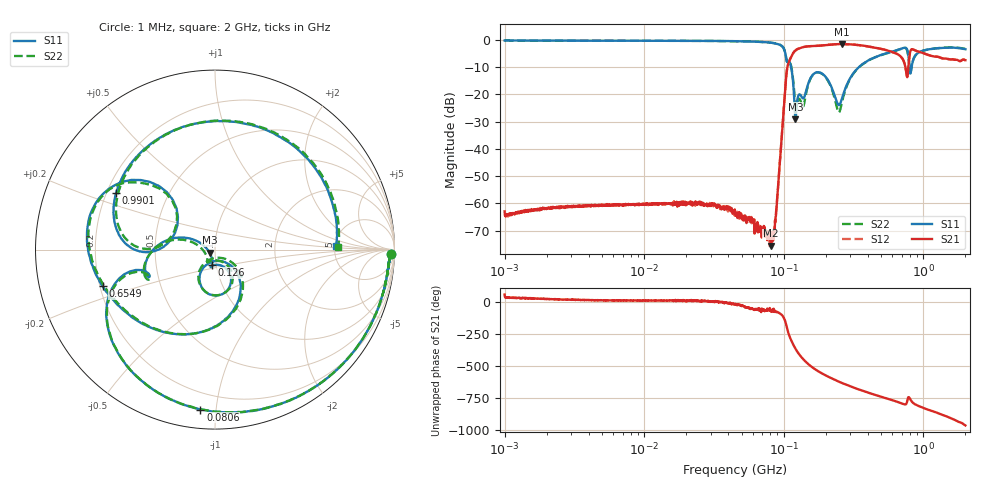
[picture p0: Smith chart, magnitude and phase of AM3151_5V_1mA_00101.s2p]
! Date/Time: Fri Jun 26 10:33:27 2020
! Network Analyzer:  Rev:
! Sweep from 1000000.0 to 2000000000.0, 1601 Points ! Power Supply: 0 V, 0 A
# HZ S DB R 50
!freq MagS11 AngS11 MagS21 AngS21 MagS12 AngS12 MagS22 AngS22
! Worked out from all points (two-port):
!   1601 points, 1 MHz to 2 GHz, reference 50 ohm
!   highest |S21| = -1.47 dB at 261.8 MHz (marker M1); lowest = -75.6 dB at 80.99 MHz (marker M2)
!   |S21| within 3 dB of the highest: 117.9 MHz to 602.8 MHz (484.9 MHz wide, 135 % of centre); 803.3 MHz to 951.4 MHz (148.1 MHz wide, 16.9 % of centre)
!   lowest |S11| = -29.2 dB at 121.3 MHz (marker M3), VSWR 1.07, Z = 47.1 - j1.64 ohm
!   |S11| at or under -10 dB: 112.9 MHz to 344.4 MHz (231.5 MHz wide, 101 % of centre); 795.6 MHz to 823.2 MHz (27.65 MHz wide, 3.42 % of centre)
!   |S22| runs from -26.6 to -0.2 dB; largest |S21 - S12| = 0.0096
!   S11 on the Smith chart (normalised r, x): 1 MHz: 37, -48; 80.6 MHz: 0.10, -0.91; 126 MHz: 0.95, -0.16; 654.9 MHz: 0.21, -0.15; 990.1 MHz: 0.24, +0.25; 2 GHz: 5.15, +0.37
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1000000  -0.17 -1.5  -62.97 59.7  -64.38 36.1  -0.17 -1.5
3555161  -0.24 -3.9  -60.89 17.4  -61.09 15.9  -0.25 -3.9
1.263916e7  -0.28 -12.7  -60.62 12.3  -60.20 12.3  -0.28 -12.7
4.493426e7  -0.43 -46.3  -63.66 -20.4  -62.81 -17.4  -0.43 -46.3
8.06017e7  -0.96 -95.2  -70.62 -68.9  -72.08 -66.7  -0.99 -95.1
8.098555e7  -0.99 -95.9  -75.59 -60.3  -74.32 -62.5  -0.99 -95.8
8.779725e7  -1.28 -109.9  -64.72 -77.8  -64.00 -72.4  -1.30 -109.7
1.051672e8  -7.85 -162.4  -11.22 162.6  -11.21 162.5  -7.81 -160.8
1.123994e8  -9.53 178.1  -6.41 66.3  -6.41 66.4  -9.15 -178.9
1.212759e8  -29.19 -150.0  -3.81 -5.8  -3.82 -5.9  -24.15 -170.7
1.259737e8  -21.19 -101.6  -3.30 -34.6  -3.30 -34.6  -22.25 -122.5
1.391892e8  -21.25 -78.8  -2.54 -92.8  -2.55 -92.7  -23.86 -72.5
1.589914e8  -13.21 -67.5  -2.23 -149.1  -2.22 -149.1  -13.28 -64.9
1.941001e8  -12.91 -108.3  -1.92 151.8  -1.90 151.8  -13.01 -109.7
2.618205e8  -21.31 -53.2  -1.47 84.5  -1.48 84.6  -22.60 -43.0
3.738861e8  -8.56 -77.6  -2.10 20.9  -2.12 20.7  -8.61 -75.5
5.652395e8  -4.62 -138.0  -4.01 -41.1  -3.99 -41.2  -4.68 -138.6
6.54923e8  -3.64 -161.9  -5.24 -63.4  -5.23 -63.4  -3.67 -163.4
8.148812e8  -11.51 172.5  -3.64 -51.7  -3.63 -51.6  -11.36 169.9
9.901099e8  -3.95 150.1  -4.75 -108.9  -4.74 -108.6  -3.99 147.1
1.441025e9  -2.85 79.4  -6.80 -173.5  -6.74 -173.4  -2.78 76.3
2e9  -3.40 1.7  -7.40 112.1  -7.55 111.8  -3.26 1.4
